FUNCTION_BLOCK ABSTRACT Substate IMPLEMENTS I_Substate
VAR
	_next : I_Substate;
END_VAR

METHOD PUBLIC IsEqual : BOOL
VAR_INPUT
	Substate : I_Substate;
END_VAR
IsEqual := Name = Substate.Name;
END_METHOD

PROPERTY PUBLIC ABSTRACT Name : T_MAXSTRING
GET
END_GET
END_PROPERTY

PROPERTY PUBLIC Next : I_Substate
GET
Next := _next;
END_GET
SET
_next := Next;
END_SET
END_PROPERTY

END_FUNCTION_BLOCK
